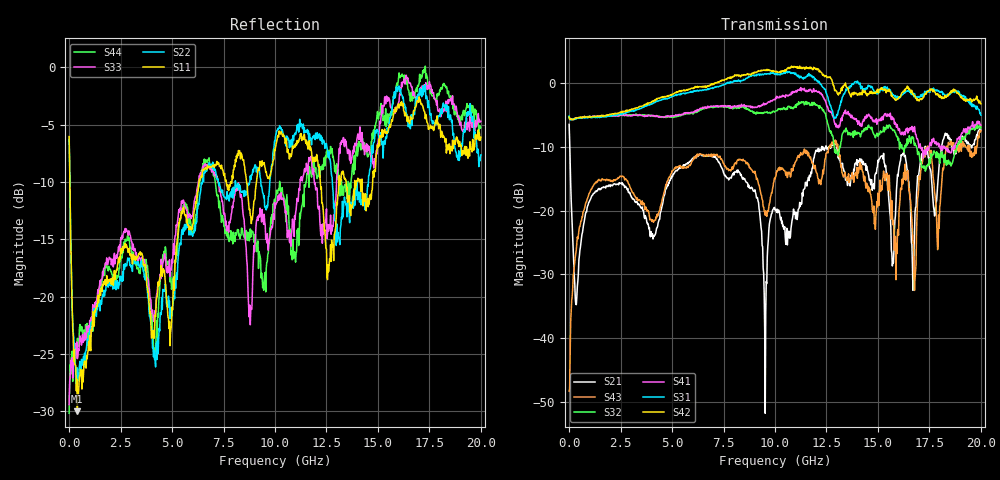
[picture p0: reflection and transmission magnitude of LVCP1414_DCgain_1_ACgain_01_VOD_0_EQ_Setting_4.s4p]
!Agilent Technologies,N5230A,MY46400459,A.07.50.48
!Agilent N5230A: A.07.50.48
!Date: Tuesday, April 17, 2012 18:46:17
!Correction: S11(Full 4 Port(1,2,3,4))
!S12(Full 4 Port(1,2,3,4))
!S13(Full 4 Port(1,2,3,4))
!S14(Full 4 Port(1,2,3,4))
!S21(Full 4 Port(1,2,3,4))
!S22(Full 4 Port(1,2,3,4))
!S23(Full 4 Port(1,2,3,4))
!S24(Full 4 Port(1,2,3,4))
!S31(Full 4 Port(1,2,3,4))
!S32(Full 4 Port(1,2,3,4))
!S33(Full 4 Port(1,2,3,4))
!S34(Full 4 Port(1,2,3,4))
!S41(Full 4 Port(1,2,3,4))
!S42(Full 4 Port(1,2,3,4))
!S43(Full 4 Port(1,2,3,4))
!S44(Full 4 Port(1,2,3,4))
!S4P File: Measurements: <S11,S12,S13,S14>,
!<S21,S22,S23,S24>,
!<S31,S32,S33,S34>,
!<S41,S42,S43,S44>:
# Hz S  dB  R 50
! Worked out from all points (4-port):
!   801 points, 300 kHz to 20 GHz, reference 50 ohm
!   strongest paths, dB at 300 kHz, 5 GHz, 10 GHz, 15 GHz, 20 GHz:
!     S42: -5.3, -1.7, 1.8, -1.0, -3.2
!     S31: -5.2, -2.1, 1.4, -1.6, -5.0
!     S41: -5.2, -5.1, -2.6, -5.8, -6.5
!     S32: -5.2, -5.3, -4.4, -8.3, -6.9
!     S43: -48.3, -13.7, -15.0, -17.2, -7.4
!     S21: -6.5, -14.5, -19.9, -12.1, -7.4
!   lowest |S11| = -30.0 dB at 400.3 MHz (marker M1), VSWR 1.07, Z = 53 + j1.26 ohm
!   |S11| at or under -10 dB: 37.27 MHz to 6.307 GHz (6.27 GHz wide, 198 % of centre); 8.621 GHz to 9.102 GHz (480.8 MHz wide, 5.43 % of centre); 12.2 GHz to 13.11 GHz (902.4 MHz wide, 7.13 % of centre)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
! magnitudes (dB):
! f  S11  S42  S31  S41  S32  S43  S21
! 300 kHz  -6.0  -5.3  -5.2  -5.2  -5.2  -48.3  -6.5
! 400.3 MHz  -30.0  -5.4  -5.4  -5.5  -5.4  -24.1  -31.9
! 6.225 GHz  -10.9  -0.5  -1.1  -4.1  -4.5  -11.1  -11.3
! 10.25 GHz  -5.8  1.9  1.3  -2.2  -4.0  -13.4  -21.1
! 12.75 GHz  -15.1  0.6  -4.1  -4.6  -7.9  -9.5  -9.8
! 16.78 GHz  -3.8  -2.0  -1.6  -6.8  -9.7  -32.5  -23.7
! 20 GHz  -6.1  -3.2  -5.0  -6.5  -6.9  -7.4  -7.4
